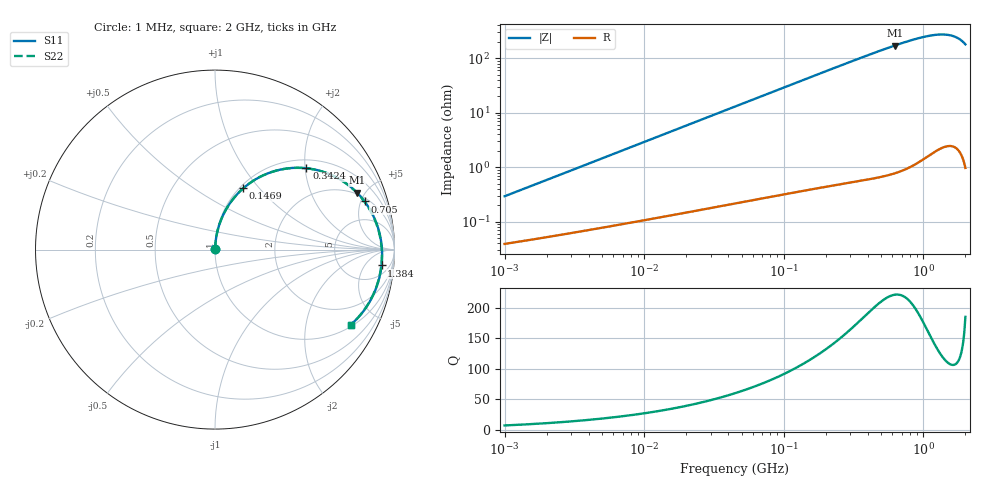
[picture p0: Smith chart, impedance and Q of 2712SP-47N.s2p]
# MHz  S  MA  R  50
!Freq  MagS11  AngS11  MagS21  AngS21  MagS12  AngS12  MagS22  AngS22
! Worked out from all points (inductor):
!   801 points, 1 MHz to 2 GHz, reference 50 ohm
!   read as one part in series: L = 46.2 nH near 1.039 MHz
!   highest Q = 222 at 623.1 MHz (marker M1), where L = 43.7 nH
!   S11 on the Smith chart (normalised r, x): 1 MHz: 1.00, +0.01; 146.9 MHz: 1.04, +0.83; 342.4 MHz: 1.20, +2.03; 705 MHz: 2.34, +5.38; 1.384 GHz: 10, -14; 2 GHz: 1.08, -3.57
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1  0.002806 81.8  0.9996 -0.2  0.9996 -0.2  0.002806 81.8
3.573795  0.009949 85.5  0.9993 -0.6  0.9993 -0.6  0.009948 85.5
12.65119  0.03512 85.9  0.9982 -2.2  0.9982 -2.2  0.03512 85.9
25.31997  0.07011 84.3  0.9959 -4.4  0.9959 -4.4  0.07009 84.3
44.78507  0.1233 81.3  0.9902 -7.7  0.9902 -7.7  0.1232 81.3
87.94465  0.2366 74.3  0.9687 -15.0  0.9687 -15.0  0.2365 74.3
114.7595  0.3026 70.1  0.9499 -19.3  0.9499 -19.3  0.3024 70.1
146.9306  0.3761 65.3  0.9231 -24.2  0.9231 -24.2  0.3758 65.3
160.0527  0.4042 63.3  0.9112 -26.1  0.9112 -26.1  0.4039 63.3
245.4796  0.559 52.1  0.8254 -37.5  0.8254 -37.5  0.5585 52.1
342.3651  0.6821 41.7  0.7276 -48.0  0.7276 -48.0  0.6814 41.7
438.3421  0.7633 33.5  0.6425 -56.2  0.6425 -56.2  0.7624 33.5
566.5845  0.8318 25.0  0.5518 -64.7  0.5518 -64.7  0.8307 25.0
623.0789  0.8524 21.9  0.5195 -67.9  0.5195 -67.9  0.8513 21.9
705.0255  0.8756 17.9  0.4797 -71.9  0.4797 -71.9  0.8744 17.8
1002.154  0.9195 6.4  0.3882 -83.3  0.3882 -83.3  0.9181 6.4
1200.504  0.9302 0.1  0.3599 -89.4  0.3599 -89.4  0.9288 0.1
1384.462  0.9322 -5.4  0.352 -94.9  0.352 -94.9  0.9308 -5.4
1551.726  0.9278 -10.6  0.3601 -100.0  0.3601 -100.0  0.9266 -10.7
1706.449  0.9172 -15.9  0.3825 -105.3  0.3825 -105.3  0.9162 -16.0
1823.846  0.9031 -20.5  0.4114 -109.9  0.4114 -109.9  0.9024 -20.5
2000  0.8647 -28.9  0.4811 -118.4  0.4811 -118.4  0.8646 -28.9
